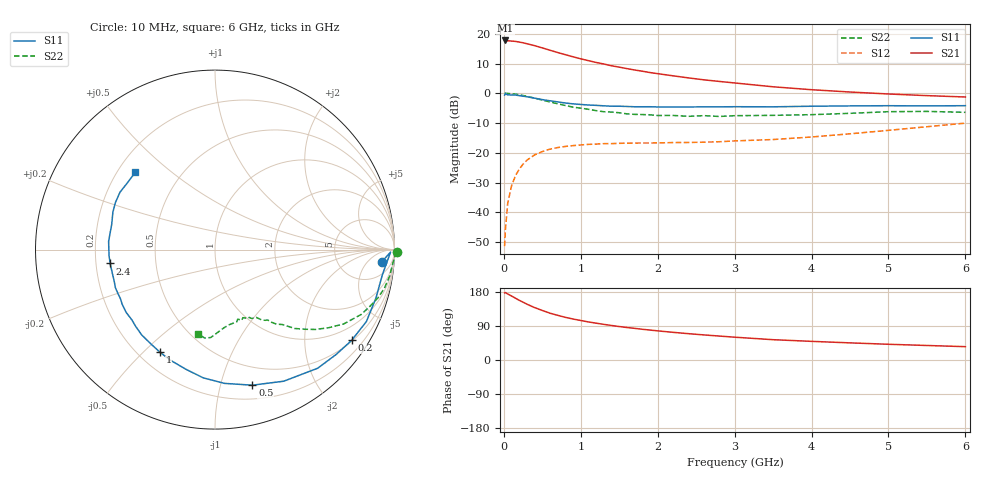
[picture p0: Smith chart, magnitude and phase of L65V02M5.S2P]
!  INFINEON TECHNOLOGIES Small Signal Semiconductors
! BFR380L3 , Si-NPN RF-Transistor in TSLP-3-1
!  Vce=5 V,  Ic=2.5 mA
! Common Emitter S-Parameters:  07. March 2005
#  GHz  S  MA  R  50
! f  S11  S21  S12  S22
! GHz  Mag  Ang  Mag  Ang  Mag  Ang  Mag  Ang
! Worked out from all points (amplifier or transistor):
!   36 points, 10 MHz to 6 GHz, reference 50 ohm
!   highest |S21| = 17.7 dB at 20 MHz (marker M1)
!   |S21| within 3 dB of that: start of sweep to 563.7 MHz
!   unconditionally stable (mu >= 1): 3.023 GHz to 4.557 GHz
!   at 250 MHz: K = 0.09, MSG = 20.4 dB, |S12| = -23.8 dB
!   at 1.4 GHz: K = 0.57, MSG = 13.1 dB, |S12| = -16.9 dB
!   at 6 GHz: K = 0.88, MSG = 4.4 dB, |S12| = -10.0 dB
!   S11 on the Smith chart (normalised r, x): 10 MHz: 14, -14; 200 MHz: 0.53, -3.23; 500 MHz: 0.32, -1.26; 1 GHz: 0.28, -0.56; 2.4 GHz: 0.26, -0.06; 6 GHz: 0.27, +0.38
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0.01  0.9329 -4.1  7.658 177.2  0.0027 89.3  1.016 -0.9
0.02  0.9784 -0.8  7.717 178.0  0.0051 91.4  1.004 -1.9
0.05  0.9429 -8.6  7.633 174.3  0.0141 88.5  0.9936 -4.4
0.1  0.9364 -16.7  7.538 168.9  0.0278 81.3  0.9842 -8.6
0.15  0.9339 -25.4  7.444 163.2  0.0409 75.8  0.9677 -12.9
0.2  0.914 -33.6  7.257 157.5  0.0532 72.6  0.9463 -16.6
0.3  0.8743 -49.1  6.798 147.3  0.0751 63.8  0.8913 -23.9
0.4  0.8273 -62.4  6.312 138.3  0.0923 57.3  0.8282 -30.0
0.5  0.7836 -74.6  5.785 130.7  0.1048 52.0  0.7684 -34.5
0.6  0.7471 -86.0  5.288 123.5  0.1152 47.3  0.7148 -38.5
0.7  0.7173 -95.3  4.836 117.9  0.1225 44.2  0.667 -41.7
0.8  0.6857 -103.8  4.453 112.6  0.1279 41.1  0.6233 -44.8
1  0.6491 -118.1  3.791 104.3  0.1354 37.4  0.562 -48.0
1.1  0.6347 -124.6  3.531 100.4  0.1385 36.1  0.5378 -50.5
1.3  0.6154 -135.8  3.103 94.0  0.1425 34.4  0.4897 -53.2
1.6  0.6002 -149.5  2.597 85.7  0.1452 33.3  0.4511 -57.9
2.2  0.587 -167.4  1.965 73.0  0.1486 36.1  0.4244 -64.4
2.4  0.5892 -172.5  1.813 69.5  0.1492 37.8  0.4099 -67.7
3.5  0.5924 166.2  1.285 53.6  0.1671 49.3  0.4258 -79.2
4.5  0.6136 154.8  1.05 45.2  0.2085 59.9  0.4604 -87.9
5.5  0.6137 142.7  0.913 38.3  0.2743 64.6  0.4961 -96.7
6  0.6189 135.7  0.866 35.2  0.315 64.5  0.4784 -101.1
